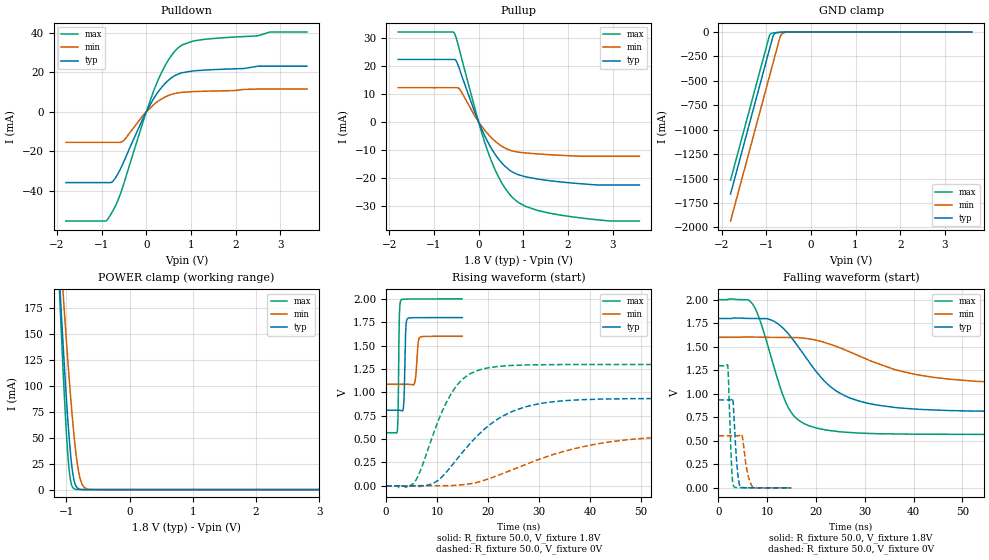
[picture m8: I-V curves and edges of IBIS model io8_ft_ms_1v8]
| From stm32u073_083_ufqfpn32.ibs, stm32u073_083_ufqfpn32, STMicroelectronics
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[Model]   io8_ft_ms_1v8
Model_type I/O
Polarity   Non-Inverting
Enable   Active-Low
| CAP_THRESHOLD on pad IOFT is "UDTCAPC" :
| Rising=30.0% of vddiom   Falling=70.0% of vddiom
| C_comp min and max val. don't necessarily correlate with the min and max pvt
| but are the smallest and greatest pad capacitance found.
| var   typ   min   max
C_comp   2.04479pF  2.03950pF  2.10328pF
|C_comp_pullup   1.14453pF  1.14099pF  1.14605pF
|C_comp_pulldown   900.25992fF  898.51017fF  957.23003fF
Vinl = 480.0mV
Vinh = 1.4V
Vmeas = 900.0mV   | Reference voltage for timing measurements
Cref  = 50.0pF   | Timing specification test load capacitance value
Rref  = 100.0MOhm   | Timing specification test load resistance value
Vref  = 900.0mV   | Timing specification test load voltage
[Model Spec]
| TIME_THRESHOLD on pin ZIV12 is "CMOS" :
| Rising=50.0% of vdd   Falling=50.0% of vdd
Vinl 728.70000mV 655.70000mV 817.70000mV
Vinh 1.06430V 949.30000mV 1.16330V
| variable   typ   min   max
[Temperature Range] 25.0 140.0 -40.0
| variable   typ   min   max
[Voltage Range] 1.8V 1.6V 2.0V
| variable   typ   min   max
[POWER Clamp Reference] 1.8V 1.6V 2.0V
| variable   typ   min   max
[GND Clamp Reference] 0V 0V 0V
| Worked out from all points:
|   slope of the pulldown table from 0 to 0.27 V, typ, clamps not added: 26.3 ohm
|   slope of the pullup table from 0 to 0.27 V, typ, clamps not added: 30 ohm
|   GND clamp passes 1 mA (typ) near -0.61 V on its own axis
|   POWER clamp passes 1 mA (typ) near -0.81 V on its own axis
|   rising waveform, R_fixture 50.0, V_fixture 1.8V: 20-80 % time 252ps typ, 396ps min, 202ps max; typ from 0.809 V to 1.8 V
|   falling waveform, R_fixture 50.0, V_fixture 1.8V: 20-80 % time 10ns typ, 17.9ns min, 5.36ns max; typ from 1.8 V to 0.809 V
|   rising waveform, R_fixture 50.0, V_fixture 0V: 20-80 % time 10.5ns typ, 18.9ns min, 6ns max; typ from 0 V to 0.935 V
|   falling waveform, R_fixture 50.0, V_fixture 0V: 20-80 % time 694ps typ, 1.02ns min, 534ps max; typ from 0.935 V to 0 V
[POWER Clamp]
-1.8V     1.053A     943.1mA    1.262A
-1.11V    202.2mA    242.3mA    190.9mA
-1.09V    180mA      223.6mA    163.4mA
-1.05V    136.9mA    187mA      110.9mA
-980mV    68.91mA    126.1mA    35.23mA
-940mV    37.57mA    94.11mA    10.65mA
-880mV    8.969mA    52.17mA    807.4uA
-830mV    1.697mA    25.82mA    75.79uA
-790mV    394.2uA    12.22mA    11.25uA
-740mV    61.25uA    3.879mA    1.034uA
-660mV    3.073uA    483.4uA    22.7nA
3.6V      0A         0A         0A
[GND Clamp]
-1.8V     -1.658A    -1.935A    -1.517A
-930mV    -179mA     -456mA     -38.91mA
-900mV    -128mA     -405mA     -17.65mA
-850mV    -44.09mA   -320mA     -9.519mA
-830mV    -24.74mA   -286mA     -8.302mA
-790mV    -9.695mA   -218mA     -6.49mA
-700mV    -2.938mA   -65mA      -3.294mA
-670mV    -2.157mA   -31.85mA   -2.435mA
-640mV    -1.545mA   -16.21mA   -1.699mA
-570mV    -571.9uA   -3.807mA   -536.5uA
-420mV    -14.26uA   -143.3uA   -5.434uA
3.6V      450.9pA    102.5nA    318pA
| variable   typ   min   max
[Pullup Reference] 1.8V 1.6V 2.0V
| variable   typ   min   max
[Pulldown Reference] 0V 0V 0V
[Pullup]
-1.8V     22.25mA    12.18mA    32.02mA
-550mV    22.25mA    12.18mA    31.76mA
-500mV    21.67mA    12.18mA    29.82mA
-420mV    18.45mA    11.57mA    25.1mA
-90mV     3.62mA     2.224mA    5.223mA
240mV     -8.143mA   -4.875mA   -12mA
540mV     -15mA      -8.867mA   -22.31mA
870mV     -18.72mA   -10.75mA   -28.48mA
1.33V     -20.4mA    -11.44mA   -31.6mA
1.9V      -21.5mA    -11.96mA   -33.39mA
2.94V     -22.49mA   -12.26mA   -35.33mA
3.6V      -22.49mA   -12.26mA   -35.33mA
[Pulldown]
-1.8V     -35.76mA   -15.41mA   -55.17mA
-910mV    -35.76mA   -15.41mA   -55.17mA
-830mV    -35.76mA   -15.41mA   -53.18mA
-710mV    -34mA      -15.41mA   -48.42mA
-520mV    -26.05mA   -14.75mA   -37.5mA
-90mV     -4.145mA   -2.306mA   -6.327mA
230mV     8.974mA    4.797mA    14.24mA
490mV     15.87mA    8.223mA    26.01mA
750mV     19.43mA    9.743mA    33.01mA
1.33V     21.16mA    10.45mA    36.75mA
2.78V     23.13mA    11.52mA    40.36mA
3.6V      23.13mA    11.52mA    40.37mA
[Ramp]
dV/dt_r 560.73079mV/10.49967ns 332.41132mV/18.91227ns 778.78265mV/5.99872ns
dV/dt_f 594.84345mV/10.00321ns 308.28301mV/17.87518ns 859.13303mV/5.36336ns
R_load = 50.0
| Removed startup time: 0s 0s 0s  .
| Removed end time: 14.9ns.
[Rising Waveform]
R_fixture   = 50.0
V_fixture   = 1.8V
V_fixture_min = 1.6V
V_fixture_max = 2.0V
0s        808.6mV    1.086V     568.1mV
2.2ns     808.7mV    1.086V     590.9mV
2.6ns     808.5mV    1.086V     1.844V
2.9ns     806.3mV    1.086V     1.985V
3.4ns     844.8mV    1.086V     1.996V
3.8ns     1.615V     1.086V     1.997V
4.1ns     1.781V     1.086V     1.998V
5.6ns     1.799V     1.104V     1.998V
6.6ns     1.799V     1.588V     1.998V
14.9ns    1.799V     1.6V       2V
| Removed startup time: 0s 0s 0s  .
| Removed end time: 199.9ns.
[Falling Waveform]
R_fixture   = 50.0
V_fixture   = 1.8V
V_fixture_min = 1.6V
V_fixture_max = 2.0V
0s        1.8V       1.6V       2V
6.9ns     1.8V       1.603V     1.96V
8.4ns     1.8V       1.601V     1.797V
11ns      1.78V      1.6V       1.352V
14.5ns    1.626V     1.6V       835.8mV
17.2ns    1.438V     1.592V     692.8mV
21.9ns    1.126V     1.543V     615.5mV
31.6ns    888.8mV    1.341V     577.2mV
52.6ns    816.1mV    1.133V     568.3mV
199.9ns   808.6mV    1.086V     568.1mV
| Removed startup time: 0s 0s 0s  .
| Removed end time: 199.9ns.
[Rising Waveform]
R_fixture   = 50.0
V_fixture   = 0V
V_fixture_min = 0V
V_fixture_max = 0V
0s        -16.13uV   -14.82uV   -10.78uV
5.3ns     -505.6uV   -209.3uV   21.35mV
6.7ns     -11.57uV   -4.395mV   160.4mV
9.2ns     24.83mV    -206.2uV   547.1mV
13.4ns    252.1mV    4.694mV    1.04V
16.7ns    468.5mV    23.45mV    1.205V
21.7ns    707.5mV    106.6mV    1.276V
31.7ns    892.5mV    315.7mV    1.296V
55.5ns    933.8mV    525.8mV    1.298V
199.9ns   934.6mV    554mV      1.298V
| Removed startup time: 0s 0s 0s  .
| Removed end time: 14.9ns.
[Falling Waveform]
R_fixture   = 50.0
V_fixture   = 0V
V_fixture_min = 0V
V_fixture_max = 0V
0s        934.6mV    554mV      1.298V
1.9ns     934.6mV    554mV      1.303V
2.7ns     941.8mV    554mV      215mV
3.1ns     832.5mV    554mV      17.99mV
3.8ns     233.2mV    553.6mV    2.473mV
4.5ns     9.753mV    562.9mV    1.587mV
4.9ns     3.126mV    544.2mV    1.418mV
6ns       1.064mV    146.3mV    1.163mV
6.9ns     798.5uV    16.14mV    1.072mV
14.9ns    352.5uV    295.5uV    166.8uV
